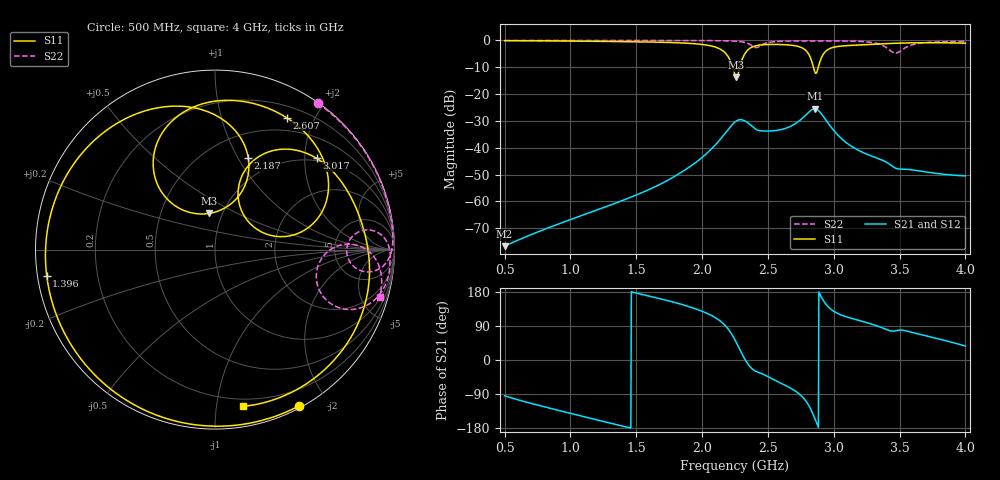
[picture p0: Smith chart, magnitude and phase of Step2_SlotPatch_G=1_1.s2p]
! TOUCHSTONE file generated by CST MICROWAVE STUDIO
! Date and time: Mon May 18 01:19:03 2020
! Project name: DualBand_DualMode_Antenna_FD_SteppedDesign.cst
! Parameters = {FPL=20; FPW=20; L=50; ST=10; SW=30; W=52; WF=7; ext=10; gap=1; inset=13}
! Header version: 2015
! Port assignment regex: !\s*Touchstone port\s*([0-9]+)\s*=\s*CST MWS port\s*([0-9]+)\s*\(\"(.*)\"\)(\s*mode\s*([0-9]+))?.*
! Touchstone port assignment:
! Touchstone port 1 = CST MWS port 1 ("")
! Touchstone port 2 = CST MWS port 2 ("")
# GHz S MA R 50
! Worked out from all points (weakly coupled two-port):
!   1006 points, 500 MHz to 4 GHz, reference 50 ohm
!   highest |S21| = -25.48 dB at 2.856 GHz (marker M1); lowest = -76.7 dB at 500 MHz (marker M2)
!   lowest |S11| = -13.8 dB at 2.26 GHz (marker M3), VSWR 1.51, Z = 43.2 + j18.2 ohm
!   |S11| at or under -10 dB: 2.232 GHz to 2.286 GHz (54.37 MHz wide, 2.41 % of centre); 2.846 GHz to 2.883 GHz (36.97 MHz wide, 1.29 % of centre)
!   |S22| runs from -4.7 to 0.0 dB; largest |S21 - S12| = 2e-05
!   S11 on the Smith chart (normalised r, x): 500 MHz: 0.02, -1.67; 1.396 GHz: 0.03, -0.08; 2.187 GHz: 0.76, +1.11; 2.607 GHz: 0.33, +1.63; 3.017 GHz: 0.94, +2.27; 4 GHz: 0.14, -1.18
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0.5  0.9886 -61.8  0.0001469 -94.3  0.0001469 -94.3  0.9965 54.9
0.787  0.9821 -97.0  0.0002925 -122.2  0.0002926 -122.2  0.9974 34.5
1.0845  0.9676 -133.5  0.0005466 -148.1  0.0005464 -148.1  0.9976 22.9
1.396  0.9488 -171.2  0.001044 -174.5  0.001043 -174.5  0.9971 15.0
1.669  0.9263 154.9  0.002018 162.8  0.002018 162.8  0.9962 9.6
2.0015  0.8395 108.2  0.006649 128.4  0.006649 128.4  0.9928 3.5
2.187  0.5444 70.1  0.02026 86.5  0.02026 86.5  0.9819 -0.9
2.25  0.2244 81.1  0.03028 52.8  0.03028 52.8  0.968 -3.1
2.2605  0.2042 99.5  0.03161 45.7  0.03161 45.7  0.9642 -3.6
2.3445  0.6531 120.7  0.02952 -8.6  0.02952 -8.7  0.8841 -7.9
2.45  0.8248 91.1  0.02063 -35.2  0.02063 -35.3  0.8104 7.1
2.607  0.8361 61.5  0.02197 -62.5  0.02197 -62.5  0.9651 1.7
2.7575  0.7305 30.0  0.03471 -95.9  0.03471 -95.9  0.9782 -2.4
2.8345  0.3968 10.6  0.05118 -136.4  0.05118 -136.4  0.9773 -4.2
2.8555  0.2614 25.2  0.05318 -153.7  0.05318 -153.7  0.977 -4.6
2.887  0.3446 68.1  0.04869 179.7  0.04869 179.7  0.9777 -5.2
2.929  0.5895 63.6  0.03599 152.8  0.03599 152.8  0.9789 -6.1
3.0165  0.7609 42.0  0.01888 125.3  0.0189 125.3  0.9778 -8.3
3.272  0.8385 6.4  0.007245 96.4  0.007243 96.4  0.9266 -18.0
3.419  0.8751 -11.0  0.005038 77.9  0.005037 78.0  0.677 -24.2
3.552  0.8969 -27.1  0.00398 76.7  0.003983 76.9  0.7479 2.3
4  0.8874 -79.9  0.002988 36.9  0.002988 36.8  0.9547 -16.2
